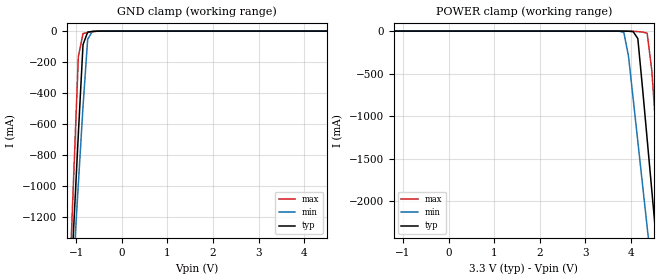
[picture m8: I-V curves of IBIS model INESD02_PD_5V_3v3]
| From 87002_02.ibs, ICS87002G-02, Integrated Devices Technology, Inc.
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[Model] INESD02_PD_5V_3v3
Model_type  Input
Polarity   Non-Inverting
Vinl = 0.8V
Vinh = 2.0V
|   typ   min   max
C_comp   2pF   1.5pF   2.5pF
|   typ   min   max
[Voltage range]  3.3V   3.15V   3.45V
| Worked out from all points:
|   GND clamp passes 1 mA (typ) near -0.58 V on its own axis
[GND_clamp]
|Voltage   I(typ)   I(min)   I(max)
-1.973V   -6.688A    -6A        -7.863A
-1.157V   -1.867A    -1.988A    -1.704A
-1.055V   -1.265A    -1.488A    -934.1mA
-952.6mV  -663.4mA   -987.4mA   -164.5mA
-850.5mV  -87.6mA    -487.5mA   -16.04mA
-748.5mV  -6.317mA   -52.72mA   -9.171mA
-646.4mV  -1.91mA    -2.66mA    -4.148mA
-340.2mV  -9.776uA   -8.593uA   -12.08uA
6.6V      128.6uA    131.6uA    121.8uA
[POWER_clamp]
|Voltage   I(typ)   I(min)   I(max)
-3.3V     128.6uA    128.3uA    124.8uA
3.64V     -9.776uA   -103.4uA   -3.241uA
3.844V    -417.5uA   -15.85mA   -26.94uA
3.946V    -1.91mA    -296.1mA   -290.3uA
4.048V    -6.317mA   -795.7mA   -1.934mA
4.151V    -87.6mA    -1.296A    -5.908mA
4.355V    -1.265A    -2.297A    -23.83mA
4.457V    -1.867A    -2.799A    -459.4mA
4.559V    -2.47A     -3.3A      -1.229A
4.661V    -3.072A    -3.801A    -1.999A
4.763V    -3.675A    -4.303A    -2.769A
5.681V    -9.099A    -8.82A     -9.698A
